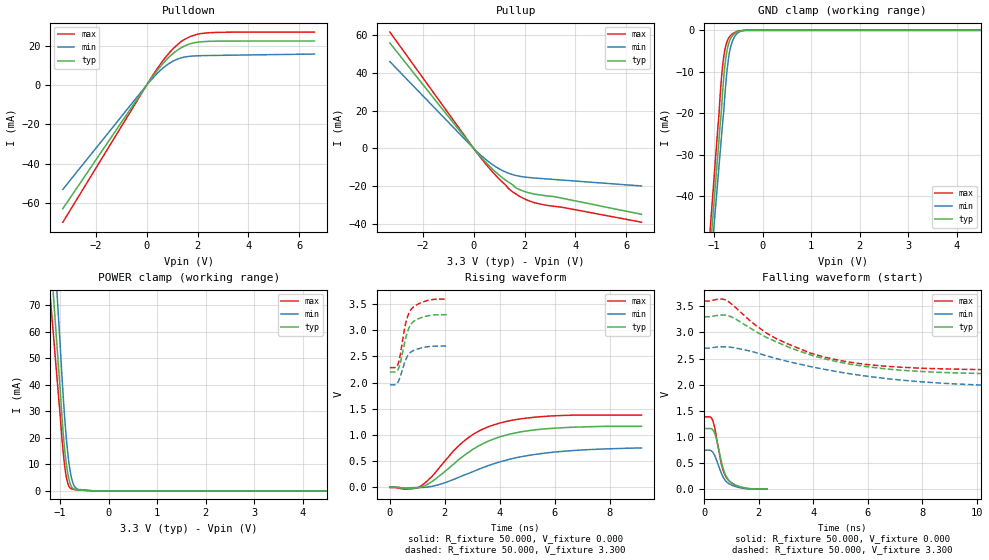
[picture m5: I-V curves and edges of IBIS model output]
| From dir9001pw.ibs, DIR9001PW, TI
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[Model]   output
Model_type Output
Vref=0.000E+00
Rref=1.000E+06
Cref=2.000E-11
Vmeas=1.650E+00
C_comp   970.0fF   970.0fF   970.0fF
[Voltage Range]   3.300E+00   2.700E+00   3.600E+00
[POWER Clamp Reference]   3.300E+00   2.700E+00   3.600E+00
[GND Clamp Reference]   0.000E+00   0.000E+00   0.000E+00
[Pullup Reference]   3.300E+00   2.700E+00   3.600E+00
[Pulldown Reference]   0.000E+00   0.000E+00   0.000E+00
[Temperature Range]   25   85   -40
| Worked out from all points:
|   slope of the pulldown table from 0 to 0.495 V, typ, clamps not added: 57 ohm
|   slope of the pullup table from 0 to 0.495 V, typ, clamps not added: 65.5 ohm
|   GND clamp passes 1 mA (typ) near -0.60 V on its own axis
|   POWER clamp passes 1 mA (typ) near -0.74 V on its own axis
|   rising waveform, R_fixture 50.000, V_fixture 0.000: 20-80 % time 1.98ns typ, 2.63ns min, 1.71ns max; typ from 0 V to 1.16 V
|   falling waveform, R_fixture 50.000, V_fixture 0.000: 20-80 % time 360ps typ, 382ps min, 349ps max; typ from 1.16 V to 0 V
|   rising waveform, R_fixture 50.000, V_fixture 3.300: 20-80 % time 326ps typ, 326ps min, 316ps max; typ from 2.2 V to 3.3 V
|   falling waveform, R_fixture 50.000, V_fixture 3.300: 20-80 % time 3.35ns typ, 4.59ns min, 2.83ns max; typ from 3.3 V to 2.2 V
[GND Clamp]
-3.3V     -382.6mA   -367.6mA   -393mA
-920mV    -29.61mA   -35.91mA   -23.26mA
-900mV    -26.67mA   -33.12mA   -20.64mA
-840mV    -17.96mA   -24.76mA   -10.57mA
-800mV    -11.43mA   -19.54mA   -6.376mA
-760mV    -6.921mA   -13.23mA   -3.817mA
-720mV    -4.133mA   -8.417mA   -2.348mA
-680mV    -2.54mA    -5.229mA   -1.518mA
-620mV    -1.31mA    -2.591mA   -863.3uA
-560mV    -644.2uA   -1.213mA   -429.9uA
-360mV    0A         0A         0A
6.6V      0A         0A         0A
[Power Clamp]
-3.3V     630.5mA    756mA      534.9mA
-1.02V    44.04mA    62.06mA    33.58mA
-940mV    23.2mA     37.52mA    15.72mA
-920mV    18.73mA    31.93mA    12mA
-880mV    11.64mA    22.16mA    6.327mA
-860mV    8.933mA    18.01mA    4.322mA
-820mV    4.72mA     11.21mA    1.873mA
-760mV    1.476mA    4.675mA    753.7uA
-720mV    783.9uA    2.341mA    572.6uA
-660mV    466.8uA    879.2uA    438uA
-260mV    0A         0A         0A
6.6V      0A         0A         0A
[Pullup]
-3.3V     55.54mA    45.75mA    61.31mA
200mV     -3.196mA   -2.613mA   -3.614mA
540mV     -8.195mA   -6.505mA   -9.29mA
880mV     -12.63mA   -9.738mA   -14.38mA
1.36V     -17.65mA   -12.99mA   -20.98mA
1.52V     -19.03mA   -13.72mA   -22.73mA
1.64V     -20.56mA   -14.15mA   -23.77mA
1.86V     -22.01mA   -14.75mA   -25.63mA
2.42V     -24.09mA   -15.58mA   -28.68mA
3.16V     -25.32mA   -16.32mA   -30.44mA
6.6V      -34.66mA   -19.74mA   -38.82mA
[Pulldown]
-3.3V     -62.95mA   -53.14mA   -69.86mA
160mV     2.986mA    2.434mA    3.346mA
580mV     10.06mA    7.967mA    11.4mA
780mV     12.91mA    10.05mA    14.71mA
1.04V     16.11mA    12.21mA    18.5mA
1.3V      18.53mA    13.62mA    21.58mA
1.64V     20.71mA    14.55mA    24.23mA
1.86V     21.48mA    14.8mA     25.36mA
2.42V     22.23mA    15.02mA    26.6mA
6.6V      22.41mA    15.77mA    26.96mA
[Rising Waveform]
R_fixture = 50.000
V_fixture = 0.000
V_fixture_min = 0.000
V_fixture_max = 0.000
|  time   V(typ)   V(min)   V(max)
0s        0V         1.292mV    -11.12mV
580ps     -26.05mV   -19.27mV   -41.3mV
1.11ns    -5.18mV    -9.546mV   12.76mV
1.54ns    106.3mV    13.43mV    207.6mV
2.33ns    443.7mV    146.9mV    699.2mV
2.77ns    629.7mV    241.7mV    910.7mV
3.27ns    797.3mV    347.9mV    1.08V
3.98ns    957.1mV    477.3mV    1.222V
5.78ns    1.119V     657.4mV    1.358V
9.16ns    1.162V     747.8mV    1.378V
[Falling Waveform]
R_fixture = 50.000
V_fixture = 0.000
V_fixture_min = 0.000
V_fixture_max = 0.000
|  time   V(typ)   V(min)   V(max)
0s        1.162V     746.6mV    1.387V
220ps     1.16V      743mV      1.38V
310ps     1.137V     707.2mV    1.314V
430ps     988.9mV    581.8mV    1.038V
640ps     494.4mV    287.6mV    451.4mV
740ps     320mV      189.3mV    292.9mV
870ps     190.2mV    116.2mV    179.9mV
1.04ns    106.9mV    69.15mV    104.7mV
1.35ns    40.77mV    23.17mV    37.15mV
2.31ns    0V         0V         0V
[Rising Waveform]
R_fixture = 50.000
V_fixture = 3.300
V_fixture_min = 2.700
V_fixture_max = 3.600
|  time   V(typ)   V(min)   V(max)
0s        2.202V     1.957V     2.286V
220ps     2.208V     1.968V     2.294V
300ps     2.252V     2.014V     2.358V
390ps     2.395V     2.13V      2.566V
480ps     2.618V     2.288V     2.869V
580ps     2.862V     2.442V     3.143V
690ps     3.04V      2.546V     3.327V
800ps     3.138V     2.598V     3.419V
1.34ns    3.273V     2.684V     3.569V
2.07ns    3.3V       2.7V       3.6V
[Falling Waveform]
R_fixture = 50.000
V_fixture = 3.300
V_fixture_min = 2.700
V_fixture_max = 3.600
|  time   V(typ)   V(min)   V(max)
0s        3.3V       2.7V       3.6V
800ps     3.329V     2.724V     3.617V
1.11ns    3.269V     2.706V     3.495V
1.85ns    3.03V      2.62V      3.15V
2.67ns    2.814V     2.497V     2.874V
3.88ns    2.573V     2.349V     2.609V
4.96ns    2.431V     2.242V     2.465V
5.97ns    2.344V     2.162V     2.386V
7.76ns    2.259V     2.064V     2.32V
12.94ns   2.202V     1.957V     2.286V
[Ramp]
dV/dt_r   6.9881E-01/1.9819E-09   4.4788E-01/2.6289E-09   8.3349E-01/1.7096E-09
dV/dt_f   6.5889E-01/3.3644E-09   4.4563E-01/4.5875E-09   7.8839E-01/2.8282E-09
R_load = 50
